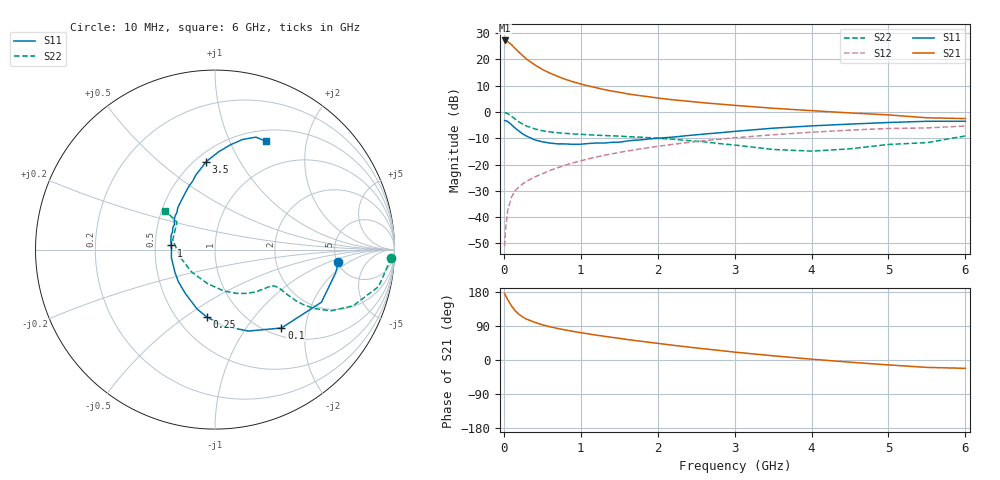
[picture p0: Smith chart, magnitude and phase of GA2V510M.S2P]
! Infineon Technologies  Discrete & RF Semiconductors
! BF775
! Si NPN RF Bipolar Junction Transistor in SOT23
! VCE = 2.5 V  IC = 10 mA
! Common Emitter S-Parameters:  May  1996
# GHz  S  MA  R  50
!  f  S11  S21  S12  S22
! GHz  MAG  ANG  MAG  ANG  MAG  ANG  MAG  ANG
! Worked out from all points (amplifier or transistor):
!   36 points, 10 MHz to 6 GHz, reference 50 ohm
!   highest |S21| = 27.2 dB at 10 MHz (marker M1)
!   |S21| within 3 dB of that: start of sweep to 145.5 MHz
!   unconditionally stable (mu >= 1): 542.1 MHz to 3.492 GHz
!   at 250 MHz: K = 0.70, MSG = 24.3 dB, |S12| = -27.3 dB
!   at 1.4 GHz: K = 1.12, MAG = 9.8 dB, |S12| = -15.9 dB
!   at 6 GHz: K = 0.97, MSG = 1.4 dB, |S12| = -5.3 dB
!   S11 on the Smith chart (normalised r, x): 10 MHz: 5.12, -1.32; 100 MHz: 1.14, -1.49; 250 MHz: 0.69, -0.61; 1 GHz: 0.61, +0.03; 3.5 GHz: 0.57, +0.73; 6 GHz: 0.63, +1.37
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0.01  0.6912 -5.6  23.02 175.7  0.0028 86.2  0.9815 -2.6
0.02  0.6849 -10.8  22.69 171.3  0.0055 85.8  0.9675 -5.2
0.05  0.6616 -26.3  21.86 159.5  0.0133 77.6  0.9348 -12.7
0.1  0.5728 -49.7  19.13 142.7  0.0241 69.2  0.8301 -22.2
0.15  0.4903 -67.7  16.04 129.4  0.0324 64.0  0.7291 -27.9
0.2  0.4304 -83.1  13.66 120.0  0.0379 62.1  0.6456 -30.6
0.25  0.3792 -96.7  11.63 112.8  0.0434 61.0  0.5814 -31.9
0.3  0.346 -106.7  10.08 107.5  0.0486 61.2  0.5369 -32.3
0.4  0.2958 -123.8  7.935 99.6  0.058 61.7  0.4787 -31.9
0.5  0.2714 -138.8  6.467 92.9  0.0668 62.8  0.4407 -31.3
0.6  0.2562 -150.9  5.489 87.7  0.0772 63.6  0.4185 -31.0
0.7  0.2479 -160.8  4.767 83.2  0.087 64.0  0.4043 -31.1
0.8  0.2472 -169.4  4.192 79.2  0.0973 63.9  0.3922 -31.4
1  0.2442 174.6  3.417 72.1  0.118 63.7  0.3757 -32.7
1.1  0.2517 168.0  3.141 68.9  0.1287 63.2  0.3695 -34.0
1.3  0.2564 157.4  2.685 62.8  0.1498 62.0  0.3574 -36.3
1.6  0.2811 143.9  2.232 54.2  0.1806 59.5  0.3409 -41.1
2.2  0.3337 123.8  1.707 38.9  0.243 53.5  0.3034 -53.5
3.5  0.4925 95.7  1.18 11.1  0.3692 37.1  0.194 -102.5
4.5  0.5898 81.7  0.962 -5.8  0.4528 23.7  0.1994 -168.2
5.5  0.6668 70.0  0.777 -19.5  0.4982 9.1  0.2613 144.1
6  0.6669 64.9  0.75 -22.0  0.5409 5.1  0.3507 142.0
